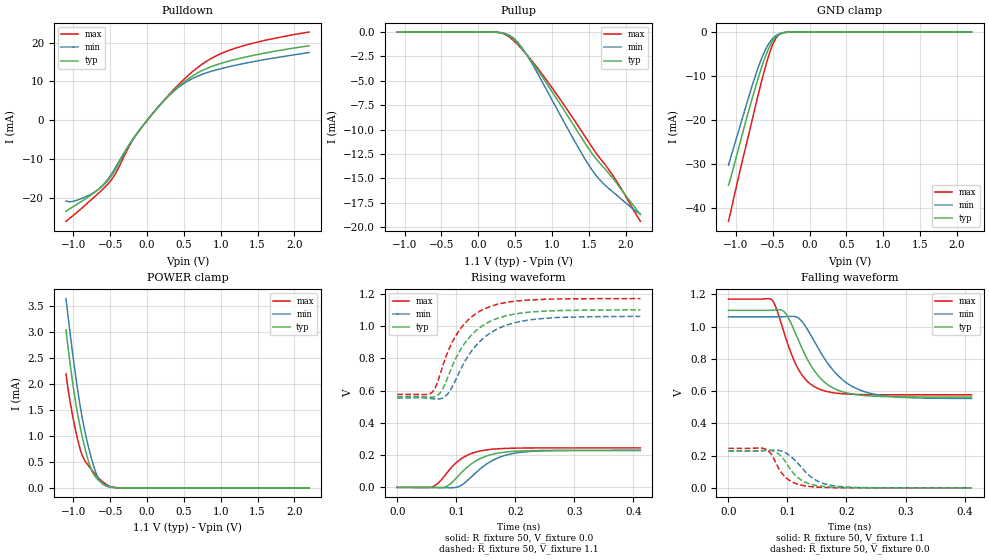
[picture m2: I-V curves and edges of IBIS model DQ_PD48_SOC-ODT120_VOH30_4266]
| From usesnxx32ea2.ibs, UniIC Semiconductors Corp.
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| DQ_PD48_SOC-ODT120_VOH30_4266
| (48 Ohm Pulldown, 120 Ohm System ODT Setting, VOH=VDDQ/3.0, 3200-4266Mbps)
[Model]   DQ_PD48_SOC-ODT120_VOH30_4266
Model_type   I/O
Vinl = 123.333mV
Vinh = 243.333mV
Vmeas = 183.333mV
Vref = 0.0mV
Cref = 0.0pF
Rref = 120.000Ohm
|   typ   min   max
|C_comp   0.834pF   0.784pF   0.884pF
C_comp_pullup   0.4170pF   0.3920pF   0.4420pF
C_comp_pulldown   0.4170pF   0.3920pF   0.4420pF
| Note: C_comp changes when the ODT circuit is enabled.
[Model Spec]
| Input threshold voltage corners
Vinl   0.1233V   0.1167V   0.1350V
Vinh   0.2433V   0.2367V   0.2550V
| Measurement voltage corners
Vmeas   0.1833V   0.1767V   0.1950V
| Timing spec test load voltage corners
Vref   0.0000V   0.0000V   0.0000V
| Dynamic Overshoot Parameters from LPDDR4 Specification
D_overshoot_ampl_h   0.30   NA   NA
D_overshoot_ampl_l   0.30   NA   NA
D_overshoot_area_h   0.1n   NA   NA
D_overshoot_area_l   0.1n   NA   NA
[Voltage Range]   1.1000V   1.0600V   1.1700V
[Pullup Reference]   1.1000V   1.0600V   1.1700V
| Junction Temperature (Ambient temp is 35C typ 95C min -40C max)
[Temperature Range]   50.0   110.0   -40.0
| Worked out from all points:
|   slope of the pulldown table from 0 to 0.165 V, typ, clamps not added: 44 ohm
|   slope of the pullup table from 0 to 0.165 V, typ, clamps not added: 38.9 kohm
|   GND clamp passes 1 mA (typ) near -0.45 V on its own axis
|   POWER clamp passes 1 mA (typ) near -0.88 V on its own axis
|   rising waveform, R_fixture 50, V_fixture 0.0: 20-80 % time 46.8ps typ, 50.9ps min, 41.7ps max; typ from 0 V to 0.23 V
|   falling waveform, R_fixture 50, V_fixture 1.1: 20-80 % time 48.8ps typ, 60.9ps min, 38.7ps max; typ from 1.1 V to 0.563 V
|   rising waveform, R_fixture 50, V_fixture 1.1: 20-80 % time 56.6ps typ, 60.8ps min, 52ps max; typ from 0.563 V to 1.1 V
|   falling waveform, R_fixture 50, V_fixture 0.0: 20-80 % time 32.2ps typ, 39.7ps min, 27.6ps max; typ from 0.23 V to 0 V
[Pulldown]
|   Voltage   I(typ)   I(min)   I(max)
-1.1V     -23.35mA   -20.65mA   -25.9mA
-1.024V   -22.39mA   -20.85mA   -24.74mA
-878.9mV  -20.68mA   -19.99mA   -22.42mA
-631.4mV  -17.27mA   -17.21mA   -18.23mA
-469.7mV  -13.86mA   -13.38mA   -14.89mA
-179.3mV  -4.509mA   -4.486mA   -4.589mA
130.9mV   2.999mA    2.977mA    3.007mA
414.7mV   8.537mA    8.295mA    8.955mA
678.7mV   12.12mA    11.31mA    13.47mA
899.8mV   14mA       12.77mA    16.22mA
1.187V    15.61mA    14.11mA    18.48mA
2.2V      19.18mA    17.44mA    22.7mA
[GND Clamp]
|   Voltage   I(typ)   I(min)   I(max)
-1.1V     -34.74mA   -30.21mA   -42.91mA
-948.2mV  -25.43mA   -21.63mA   -31.79mA
-789.8mV  -15.72mA   -12.78mA   -20.72mA
-720.5mV  -11.75mA   -9.185mA   -15.87mA
-661.1mV  -8.566mA   -6.435mA   -11.85mA
-588.5mV  -5.114mA   -3.681mA   -7.298mA
-519.2mV  -2.564mA   -1.833mA   -3.66mA
-469.7mV  -1.358mA   -991.2uA   -1.787mA
-413.6mV  -565uA     -420.4uA   -620.8uA
-350.9mV  -166uA     -126.7uA   -146.9uA
-228.8mV  -6.698uA   -6.444uA   -3.568uA
2.2V      0A         0A         0A
[Pullup]
|   Voltage   I(typ)   I(min)   I(max)
-1.1V     2.092uA    3.225uA    943.3nA
229.9mV   -15.11uA   -15.29uA   -15.56uA
332.2mV   -107.7uA   -90.15uA   -148.1uA
437.8mV   -483.6uA   -396.5uA   -608.7uA
546.7mV   -1.257mA   -1.152mA   -1.37mA
678.7mV   -2.516mA   -2.582mA   -2.496mA
1.042V    -6.565mA   -7.519mA   -6.134mA
1.388V    -10.66mA   -12.23mA   -9.986mA
1.566V    -12.67mA   -14.36mA   -12.04mA
1.688V    -13.75mA   -15.45mA   -13.26mA
1.867V    -15.37mA   -16.63mA   -15.15mA
2.2V      -18.72mA   -18.62mA   -19.39mA
[POWER Clamp]
|   Voltage   I(typ)   I(min)   I(max)
-1.1V     3.033mA    3.633mA    2.184mA
-1.041V   2.345mA    2.929mA    1.625mA
-977.9mV  1.723mA    2.241mA    1.16mA
-908.6mV  1.178mA    1.582mA    748uA
-852.5mV  818.6uA    1.148mA    543.6uA
-786.5mV  476.4uA    738.2uA    408.6uA
-737mV    296.5uA    478.3uA    318.4uA
-671mV    164.5uA    215.8uA    210.2uA
-598.4mV  83.69uA    71.97uA    113uA
-496.1mV  20.09uA    12.36uA    25.7uA
-387.2mV  1.884uA    1.296uA    1.609uA
2.2V      0A         0A         0A
[Ramp]
|   typ   min   max
| 20% - 80%
dV/dt_r   137.79m/46.76p   137.34m/50.87p   146.98m/41.66p
dV/dt_f   322.26m/48.81p   303.44m/60.92p   355.99m/38.75p
| 25% - 75%
|dV/dt_r   114.82m/37.28p   114.45m/40.63p   122.48m/33.07p
|dV/dt_f   268.55m/38.94p   252.87m/48.64p   296.66m/30.86p
R_load = 50
[Rising Waveform]
R_fixture = 50
V_fixture = 0.0
|   Time   V(typ)   V(min)   V(max)
0s        194.6uV    153.1uV    147.7uV
59ps      -158.9uV   377.3uV    2.635mV
70ps      -1.547mV   -498.2uV   29.23mV
81ps      2.941mV    -1.786mV   76.01mV
108ps     88.68mV    12.4mV     176.7mV
128ps     151.9mV    73.89mV    213.5mV
147ps     188.8mV    133.8mV    230.4mV
176ps     215.8mV    190.6mV    240.7mV
214ps     226.7mV    219.4mV    244.2mV
412ps     229.8mV    229.1mV    245.1mV
[Falling Waveform]
R_fixture   = 50
V_fixture   = 1.1
V_fixture_min = 1.06
V_fixture_max = 1.17
|   Time   V(typ)   V(min)   V(max)
0s        1.1V       1.06V      1.17V
73ps      1.101V     1.06V      1.167V
81ps      1.103V     1.06V      1.113V
94ps      1.093V     1.061V     964.7mV
117ps     927.7mV    1.056V     744.7mV
135ps     788mV      974.8mV    655.7mV
156ps     678.6mV    840.5mV    609mV
192ps     597.1mV    674.2mV    583.6mV
233ps     571.4mV    593.2mV    577.9mV
412ps     562.9mV    554.3mV    576.7mV
[Rising Waveform]
R_fixture   = 50
V_fixture   = 1.1
V_fixture_min = 1.06
V_fixture_max = 1.17
|   Time   V(typ)   V(min)   V(max)
0s        562.7mV    553.9mV    576.6mV
58ps      559.1mV    550mV      586.4mV
66ps      565.6mV    547.5mV    629.6mV
80ps      632.4mV    560.2mV    785.5mV
95ps      767.2mV    635.2mV    912.4mV
113ps     886.4mV    770.9mV    1.01V
153ps     1.02V      945.1mV    1.115V
183ps     1.062V     1.003V     1.145V
228ps     1.087V     1.04V      1.162V
412ps     1.1V       1.06V      1.17V
[Falling Waveform]
R_fixture = 50
V_fixture = 0.0
|   Time   V(typ)   V(min)   V(max)
0s        229.9mV    229.2mV    245.2mV
60ps      232.7mV    230.1mV    244mV
70ps      232.6mV    233mV      220.4mV
78ps      225.5mV    234.2mV    171.6mV
98ps      153.2mV    214.6mV    61.21mV
113ps     79.1mV     170mV      28.43mV
130ps     35.4mV     101.3mV    12.07mV
154ps     11.58mV    36.65mV    3.717mV
186ps     2.841mV    9.147mV    890uV
412ps     263.4uV    252.2uV    168.7uV
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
